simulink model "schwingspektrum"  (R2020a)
settings: Solver=ode45  StartTime=0.0  StopTime=100  RelTol=1e-3  EnableMultiTasking=on
libraries: simulink_extras x2

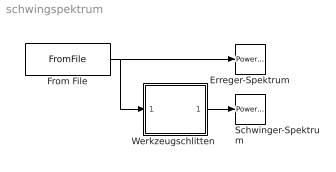
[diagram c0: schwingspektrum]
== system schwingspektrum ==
  Erreger-Spektrum : simulink_extras/Additional Sinks/Power Spectral Density  npts=1024  fftpts=1024  HowOften=64  sampleT=0.05
  From File : FromFile  FileName=schwingung.mat  SampleTime=0
  Schwinger-Spektrum : simulink_extras/Additional Sinks/Power Spectral Density  npts=1024  fftpts=1024  HowOften=64  sampleT=0.05
  "Werkzeugschlitten " : Subsystem  mask(Schwingkreis){D=0.001, om0=50, b0=40}
      mask prompts: D "Daempfungsgrad"; om0 "Eigenfrequenz"; b0 "Staerke"
      mask help: Harmonischer Schwinger mit Eigenfrequenz omega0 und Daempfungsgrad D. Die Erregerfunktion werde mit einer Verstaerkung eingekoppelt.
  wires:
  From File/1 -> "Werkzeugschlitten "/1(u), Erreger-Spektrum/1
  "Werkzeugschlitten "/1(x) -> Schwinger-Spektrum/1

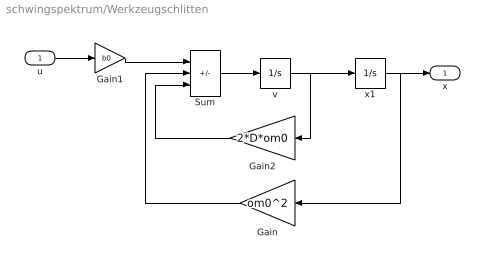
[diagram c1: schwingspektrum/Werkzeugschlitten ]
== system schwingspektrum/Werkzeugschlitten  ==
  u : Inport
  Gain : Gain  Gain=om0^2  SaturateOnIntegerOverflow=on
  Gain1 : Gain  Gain=b0  SaturateOnIntegerOverflow=on
  Gain2 : Gain  Gain=2*D*om0  SaturateOnIntegerOverflow=on
  Sum : Sum  Inputs=+--  SaturateOnIntegerOverflow=on
  v : Integrator
  x1 : Integrator
  x : Outport
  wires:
  Gain/1 -> Sum/2
  Gain2/1 -> Sum/3
  u/1 -> Gain1/1
  x1/1 -> Gain/1, x/1
  Gain1/1 -> Sum/1
  v/1 -> Gain2/1, x1/1
  Sum/1 -> v/1
